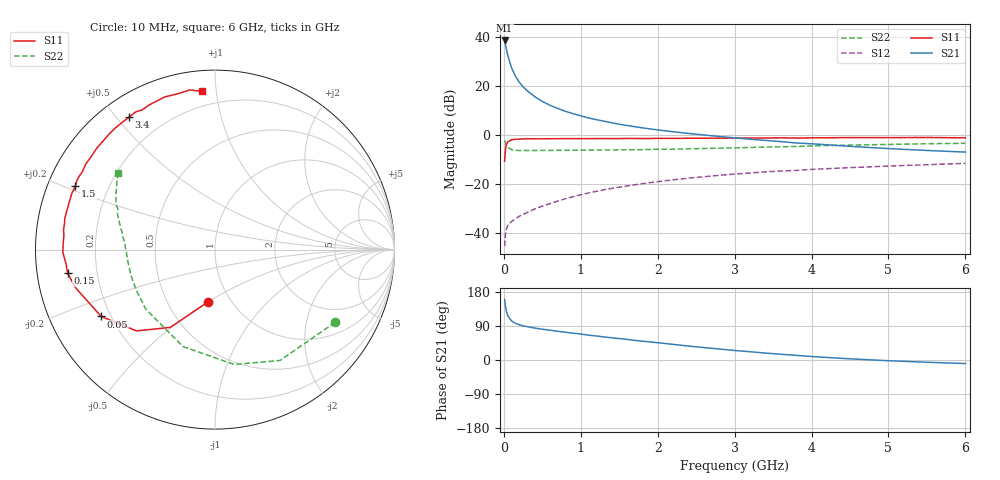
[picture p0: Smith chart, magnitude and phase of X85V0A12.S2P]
! SIEMENS Small Signal Semiconductors
! BFP136W
! Si NPN RF Bipolar Junction Transistor in SOT343
! VCE = 5 V  IC = 120 mA
! Common Emitter S-Parameters:  September  1994
# GHz  S  MA  R  50
!  f  S11  S21  S12  S22
! GHz  MAG  ANG  MAG  ANG  MAG  ANG  MAG  ANG
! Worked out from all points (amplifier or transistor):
!   40 points, 10 MHz to 6 GHz, reference 50 ohm
!   highest |S21| = 38.6 dB at 10 MHz (marker M1)
!   |S21| within 3 dB of that: start of sweep to 30.33 MHz
!   unconditionally stable (mu >= 1): 522.5 MHz to 2.989 GHz; 3.076 GHz to 3.219 GHz; 3.781 GHz to 3.82 GHz
!   at 200 MHz: K = 0.70, MSG = 27.3 dB, |S12| = -33.0 dB
!   at 1.5 GHz: K = 1.11, MAG = 10.8 dB, |S12| = -21.2 dB
!   at 6 GHz: K = 0.97, MSG = 2.3 dB, |S12| = -11.5 dB
!   S11 on the Smith chart (normalised r, x): 10 MHz: 0.78, -0.50; 50 MHz: 0.16, -0.26; 150 MHz: 0.09, -0.08; 1.5 GHz: 0.08, +0.22; 3.4 GHz: 0.08, +0.54; 6 GHz: 0.11, +0.92
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0.01  0.2956 -97.9  85.3 159.6  0.0055 68.8  0.7825 -31.2
0.02  0.4999 -119.9  72.45 142.8  0.0092 55.6  0.716 -59.6
0.03  0.6297 -134.0  60.74 131.1  0.0119 47.5  0.649 -80.5
0.05  0.7354 -149.6  42.96 117.2  0.0145 38.4  0.5689 -108.2
0.1  0.8055 -164.7  23.63 103.1  0.0175 36.6  0.5086 -139.3
0.15  0.8318 -170.9  16.06 96.9  0.0198 40.6  0.4936 -152.1
0.2  0.8333 -174.4  12.06 93.0  0.0224 42.6  0.4898 -159.0
0.25  0.841 -177.1  9.729 90.2  0.0244 44.7  0.4894 -163.4
0.3  0.8481 -179.0  8.138 88.2  0.0265 47.7  0.4884 -166.4
0.4  0.8462 177.2  6.129 84.3  0.0315 51.2  0.4891 -170.4
0.5  0.8456 174.5  4.887 81.2  0.036 54.3  0.4901 -173.2
0.6  0.8511 172.6  4.079 78.7  0.0404 56.5  0.4907 -175.0
0.7  0.8512 170.1  3.518 75.7  0.0456 58.3  0.4925 -176.3
0.9  0.8538 166.4  2.749 70.8  0.0559 59.7  0.494 -178.9
1.1  0.854 162.1  2.251 65.5  0.0666 60.3  0.4975 179.4
1.5  0.8553 155.4  1.678 56.6  0.0875 59.6  0.5032 176.3
2.2  0.8625 143.1  1.178 41.3  0.1235 54.8  0.521 170.9
3.2  0.8768 126.2  0.83 21.8  0.1702 45.5  0.5627 162.2
3.4  0.8794 123.1  0.786 18.3  0.1796 43.3  0.5756 160.5
4.5  0.8952 108.2  0.595 3.1  0.219 33.5  0.6309 151.0
5.5  0.9006 99.0  0.49 -6.0  0.2513 25.5  0.671 144.5
6  0.8847 94.6  0.454 -9.3  0.2676 21.3  0.6861 141.7
